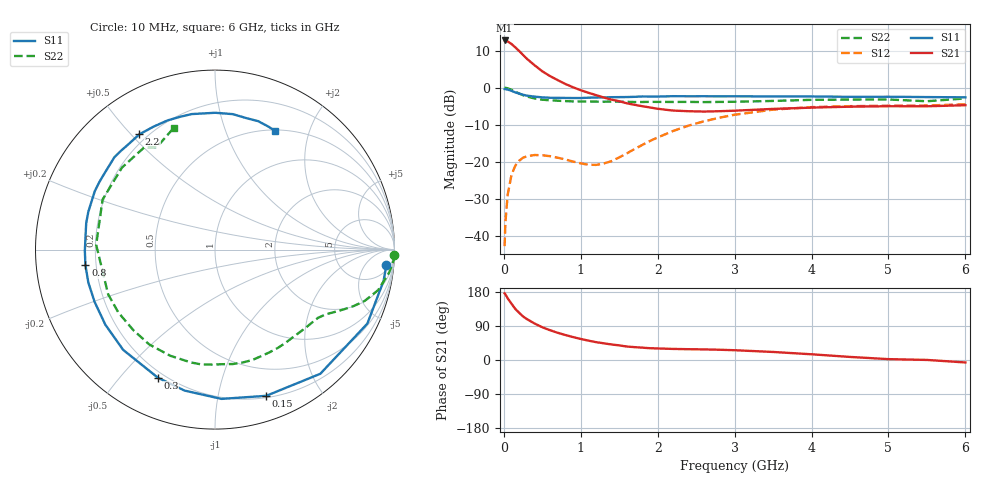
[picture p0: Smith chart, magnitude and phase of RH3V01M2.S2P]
! SIEMENS Small Signal Semiconductors
! BFR106
! Si NPN RF Bipolar Junction Transistor in SOT23
! VCE = 3 V  IC = 1.2 mA
! Common Emitter S-Parameters:  August  1996
# GHz  S  MA  R  50
!  f  S11  S21  S12  S22
! GHz  MAG  ANG  MAG  ANG  MAG  ANG  MAG  ANG
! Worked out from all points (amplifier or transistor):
!   36 points, 10 MHz to 6 GHz, reference 50 ohm
!   highest |S21| = 12.8 dB at 10 MHz (marker M1)
!   |S21| within 3 dB of that: start of sweep to 206.3 MHz
!   unconditionally stable (mu >= 1): 849.6 MHz to 2.128 GHz; 2.544 GHz to end of sweep
!   at 250 MHz: K = 0.28, MSG = 13.9 dB, |S12| = -18.9 dB
!   at 1.4 GHz: K = 1.40, MAG = 4.5 dB, |S12| = -19.8 dB
!   at 6 GHz: K = 1.02, MAG = -1.0 dB, |S12| = -4.5 dB
!   S11 on the Smith chart (normalised r, x): 10 MHz: 8, -18; 150 MHz: 0.22, -1.39; 300 MHz: 0.17, -0.63; 800 MHz: 0.16, -0.06; 2.2 GHz: 0.17, +0.53; 6 GHz: 0.51, +1.50
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0.01  0.9585 -5.3  4.355 176.0  0.0072 88.9  0.9991 -1.6
0.02  0.9553 -10.5  4.344 173.4  0.0149 84.5  0.9986 -3.1
0.05  0.9437 -25.9  4.224 162.8  0.0359 75.4  0.9787 -7.5
0.1  0.9072 -49.7  3.9 148.5  0.0667 63.0  0.937 -13.9
0.15  0.8632 -70.7  3.504 134.5  0.0887 51.3  0.8817 -18.9
0.2  0.8326 -87.5  3.131 124.4  0.1031 43.5  0.8335 -22.2
0.25  0.8036 -102.2  2.77 114.9  0.1131 36.3  0.7908 -24.9
0.3  0.7812 -114.1  2.46 107.9  0.1184 31.7  0.7609 -26.9
0.4  0.7575 -132.5  2.009 96.2  0.1231 24.3  0.715 -30.3
0.5  0.7405 -145.6  1.666 86.4  0.1221 19.6  0.6886 -33.5
0.6  0.7313 -156.6  1.437 78.6  0.1186 17.1  0.6762 -37.0
0.8  0.7271 -173.1  1.123 65.9  0.1071 17.5  0.6587 -44.6
1.1  0.7326 168.4  0.854 51.1  0.0909 31.2  0.65 -57.4
1.3  0.7384 158.5  0.737 44.0  0.0945 47.7  0.6469 -66.6
1.6  0.7479 145.6  0.615 35.5  0.1297 66.3  0.6453 -81.1
2.2  0.7683 123.3  0.491 29.2  0.2599 68.2  0.6418 -112.9
2.8  0.7651 104.8  0.481 27.1  0.3926 54.5  0.6424 -146.9
3.5  0.7623 89.9  0.517 21.2  0.5051 36.5  0.6625 177.7
4.5  0.753 76.5  0.554 8.1  0.5634 14.7  0.691 138.6
5  0.7549 71.4  0.562 2.3  0.5706 6.7  0.693 124.5
5.5  0.747 66.5  0.561 0.2  0.5746 3.0  0.6564 119.6
6  0.7415 63.3  0.58 -6.5  0.5969 -4.7  0.7162 108.7
